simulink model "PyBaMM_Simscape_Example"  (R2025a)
settings: Solver=VariableStepAuto  StartTime=0.0  StopTime=3600*2  FixedStep=0.1  RelTol=1e-3
undefined symbols (not defined in the file or in its folder): BatteryCurrent
libraries: fl_lib x3, batt_lib x1, ee_lib x1, nesl_utility x1

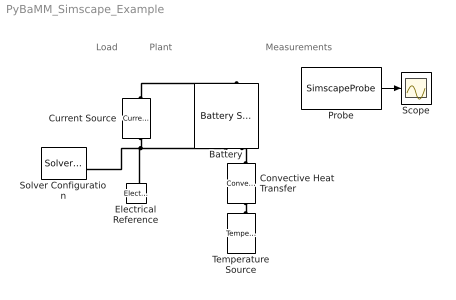
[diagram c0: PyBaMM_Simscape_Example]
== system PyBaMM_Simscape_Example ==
  note: Plant
  note: Load
  note: Measurements
  Battery : batt_lib/Cells/Electrochemical/Battery Single Particle  ExtrapolationMethod=simscape.enum.extrapolation.nearest  ThicknessAnode=8.52e-05 m  ElectrolyteLayerCountAnode=20  ThicknessSeparator=1.2e-05 m  ElectrolyteLayerCountSeparator=20  ThicknessCathode=7.56e-05 m  ElectrolyteLayerCountCathode=20  ElectrodePlateArea=0.1027 m^2  ParticleRadiusAnode=5.86e-06 m  ShellCountAnode=20  ParticleRadiusCathode=5.22e-06 m  ShellCountCathode=20  ActiveMaterialVolumeFractionAnode=0.75  ActiveMaterialVolumeFractionCathode=0.665  StoichiometryBreakpointsSpecification=simscape.battery.enum.cells.electrochemical.StoichiometryBreakpointsSpecification.normalized  NormalizedStoichiometryBreakpoints=[0,0.034483,0.068966,0.10345,0.13793,0.17241,0.2069,0.24138,0.27586,0.31034,0.34483,0.37931,0.41379,0.44828,0.48276,0.51724,0.55172,0.58621,0.62069,0.65517,0.68966,0.72414,0.75862,0.7931,0.82759,0.86207,0.89655,0.93103,0.96552,1]  OpenCircuitPotentialAnode=[1.1075,0.57004,0.43716,0.33811,0.25594,0.22015,0.21536,0.20245,0.17802,0.16196,0.1495,0.13932,0.13507,0.13283,0.13261,0.13264,0.13201,0.13201,0.12976,0.11293,0.098564,0.094697,0.09344,0.092486,0.092827,0.091811,0.091876,0.091101,0.090597,0.084577] V  OpenCircuitPotentialCathode=[4.2846,4.2294,4.1981,4.1873,4.1775,4.156,4.1254,4.0928,4.0624,4.0353,4.0105,3.9865,3.9612,3.9326,3.9008,3.8682,3.8386,3.8135,3.7922,3.7733,3.7557,3.7387,3.7221,3.7056,3.6892,3.6729,3.6565,3.6402,3.6239,3.6075] V  AbsoluteStoichiometryBreakpointsAnode=linspace(0.025, 0.975, 39)  OpenCircuitPotentialAbsoluteAnode=[.484; .335; .253; .209; .2; .181; .165; .151; .139; .131; .128; .125; .124; .124; .123; .122; .119; .117; .111; .108; .101; .098; .095; .093; .092; .088; .088; .088; .088; .087; .087; .087; .085; .082; .079; .071; .064; .049; .026] V  AbsoluteStoichiometryBreakpointsCathode=linspace(0.025, 0.975, 39)  OpenCircuitPotentialAbsoluteCathode=[3.81; 3.608; 3.512; 3.478; 3.459; 3.453; 3.45257; 3.45214; 3.45171; 3.45128; 3.45085; 3.45042; 3.44999; 3.44956; 3.44913; 3.4487; 3.44827; 3.44784; 3.44741; 3.44698; 3.44655; 3.44612; 3.44569; 3.44526; 3.44483; 3.4444; 3.44397; 3.44354; 3.44311; 3.44268; 3.44225; 3.44182; 3.44139; 3.44096; 3.44053; 3.44; 3.412; 3.304; 2.968] V  MaximumConcentrationAnode=33133 mol/m^3  MaximumStoichiometryAnode=0.90706  MinimumStoichiometryAnode=0.03022  MaximumConcentrationCathode=63104 mol/m^3  MaximumStoichiometryCathode=0.85139  MinimumStoichiometryCathode=0.26622  ActiveMaterialDiffusionCoefficientAnode=3.3e-14 m^2/s  ActiveMaterialDiffusionCoefficientCathode=4e-15 m^2/s  ConductivityAnode=215 S/m  ConductivityCathode=0.18 S/m  CurrentCollectorResistance=6.2208e-12 Ohm  ElectrolyteVolumeFractionAnode=0.25  ElectrolyteVolumeFractionSeparator=0.47  ElectrolyteVolumeFractionCathode=0.335  ElectrolyteConductivity=0.9487 S/m  BruggemanExponentAnode=1.5  BruggemanExponentSeparator=1.5  BruggemanExponentCathode=1.5  TransferenceNumber=0.2594  ElectrolyteDiffusionCoefficient=1.7694e-10 m^2/s  ChargeTransferRateAnode=6.716e-12 m^(5/2)/(mol^(1/2)*s)  ChargeTransferRateCathode=3.5446e-11 m^(5/2)/(mol^(1/2)*s)  BatteryThermalMass=42.7753 J/K  ArrheniusReferenceTemperature=298.15 K  ActiveMaterialDiffusionActivationEnergyAnode=30300.1362 J/mol  ActiveMaterialDiffusionActivationEnergyCathode=25000.1124 J/mol  ElectrolyteDiffusionActivationEnergy=17000.0764 J/mol  ConductivityActivationEnergyAnode=3000 J/mol  ConductivityActivationEnergyCathode=3000 J/mol  ElectrolyteConductivityActivationEnergy=17000.0764 J/mol  ChargeTransferActivationEnergyAnode=35000.1574 J/mol  ChargeTransferActivationEnergyCathode=17800.08 J/mol  batteryCurrent_specify=off  batteryCurrent_priority=None  batteryCurrent=0 A  batteryCurrent_nominal_specify=off  batteryCurrent_nominal_value=1  batteryCurrent_nominal_unit=A  batteryVoltage_specify=off  batteryVoltage_priority=None  batteryVoltage=0 V  batteryVoltage_nominal_specify=off  batteryVoltage_nominal_value=1  batteryVoltage_nominal_unit=V  averageElectrolyteConcentration_specify=on  averageElectrolyteConcentration_priority=High  averageElectrolyteConcentration=1000 mol/m^3  averageElectrolyteConcentration_nominal_specify=off  averageElectrolyteConcentration_nominal_value=1  averageElectrolyteConcentration_nominal_unit=mol/m^3  stateOfCharge_specify=on  stateOfCharge_priority=High  stateOfCharge=1  stateOfCharge_nominal_specify=off  stateOfCharge_nominal_value=1  stateOfCharge_nominal_unit=1  batteryTemperature_specify=on  batteryTemperature_priority=High  batteryTemperature=298.15 K  batteryTemperature_nominal_specify=off  batteryTemperature_nominal_value=1  batteryTemperature_nominal_unit=K  power_dissipated_specify=off  power_dissipated_priority=None  power_dissipated=0 W  power_dissipated_nominal_specify=off  power_dissipated_nominal_value=1  power_dissipated_nominal_unit=W  heatGenerationRate_specify=off  heatGenerationRate_priority=None  heatGenerationRate=0 W  heatGenerationRate_nominal_specify=off  heatGenerationRate_nominal_value=1  heatGenerationRate_nominal_unit=W
  Convective Heat Transfer : fl_lib/Thermal/Thermal Elements/Convective Heat Transfer  thermal_type=foundation.enum.constant_variable.constant  area=CoolingSurfaceArea m^2  heat_tr_coeff=HeatTransferCoefficient W/(K*m^2)  min_heat_tr_coeff=1e-3 W/(K*m^2)  T_specify=off  T_priority=None  T=0 K  T_nominal_specify=off  T_nominal_value=1  T_nominal_unit=K  Q_specify=off  Q_priority=None  Q=0 W  Q_nominal_specify=off  Q_nominal_value=1  Q_nominal_unit=W
  Current Source : ee_lib/Sources/Current Source  dc_current=-BatteryCurrent A  ac_current=0 A  ac_shift=0 rad  ac_frequency=60 Hz  noise_mode=ee.enum.sources.noise.Disabled  PSD=0 A^2/Hz  sample_time=1e-3 s  repeatability=ee.enum.sources.repeatability.NotRepeatable  user_seed=0  auto_seed=3046698749  i_specify=off  i_priority=None  i=0 A  i_nominal_specify=off  i_nominal_value=1  i_nominal_unit=A  v_specify=off  v_priority=None  v=0 V  v_nominal_specify=off  v_nominal_value=1  v_nominal_unit=V
  Electrical Reference : fl_lib/Electrical/Electrical Elements/Electrical Reference
  Probe : SimscapeProbe  BoundBlock=5  Variables="{\"batteryVoltage\":{\"Probing\":\"ON\"}}"
  Scope : Scope
  Solver Configuration : nesl_utility/Solver Configuration  PhysicalDomain=network_engine_domain  SubClassName=solver  LeftPortType=input  RightPortType=generic  Tones=[]  Harmonics=[]  SimulateNoise=off  Profile=off  UseLocalSampling=off  EnableSwitchedLinearOptims=on  FrequencyDomain=off  UseCCode=off  RelTol=0.001  AbsTol=0.001  MinStep=1e-09  ToWorkspace=off  RevertToSquareIcSolve=off  NumHomotopyIterations=100  PhasorMode=off  PhasorModeNumHarmonics=1  ConsistencySolver=NEWTON_XTOL_AFTER_FTOL  IndexReductionMethod=DerivativeReplacement  DoDC=off  ResidualTolerance=1e-09  ConsistencyTolSource=GLOBAL  ConsistencyAbsTol=0.001  ConsistencyRelTol=0.001  ConsistencyTolFactor=0.001  UseLocalSolver=off  LocalSolverChoice=NE_BACKWARD_EULER_ADVANCER  ResolveIndetEquations=on  FunctionEvalNumThread=1  LocalSolverSampleTime=0.001  DoFixedCost=off  MaxNonlinIter=3  MaxModeIter=2  ComputeImpulses=off  ImpulseIterations=2  LinearAlgebra=auto  LinearAlgebraNumThread=0  EquationFormulation=NE_TIME_EF  DelaysMemoryBudget=1024  AutomaticFiltering=on  FilteringTimeConstant=0.001  PartitionStorageMethod=AS_NEEDED  PartitionMemoryBudget=1024  PartitionMethod=ROBUST  MultibodyUseLocalSolver=off  MultibodyLocalSolverChoice=ODE1  MultibodyLocalSolverSampleTime=0.001
  Temperature Source : fl_lib/Thermal/Thermal Sources/Temperature Source  temperature=AmbientTemperature K
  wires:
  Probe/1 -> Scope/1
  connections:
  Convective Heat Transfer/LConn1 -- Battery/RConn2
  Temperature Source/LConn1 -- Convective Heat Transfer/RConn1
  Current Source/LConn1 -- Battery/LConn1
  Current Source/RConn1 -- Solver Configuration/RConn1 -- Electrical Reference/LConn1 -- Battery/RConn1
